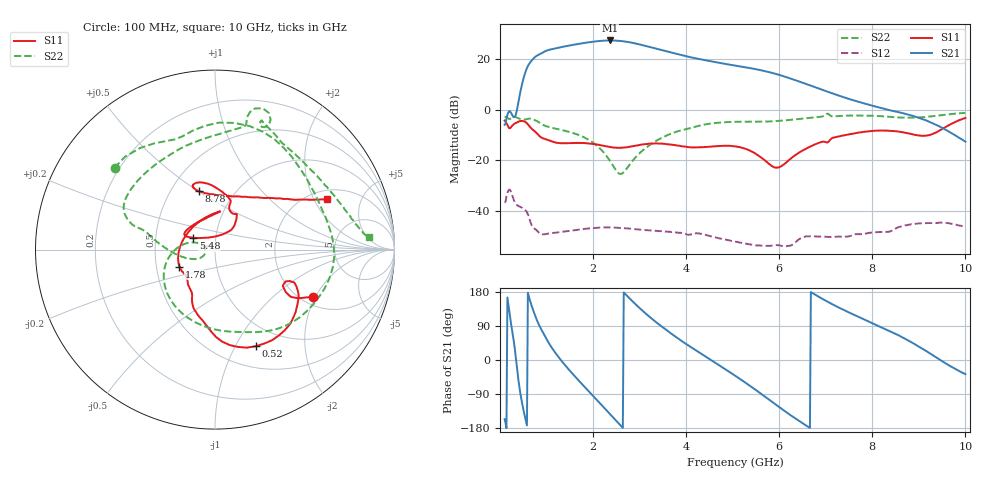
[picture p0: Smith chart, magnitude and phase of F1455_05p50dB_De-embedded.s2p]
! Integrated Device Technology
! Corporate Headquarters
! 6024 Silver Creek Valley Road
! San Jose, CA 95138  USA
! Phone:  1-408-284-8200
! Toll Free:  1-800-223-1366
! Webpage:  http://www.idt.com/
! Timing and RF Division
! 515 Groton Road, Suite 102
! Westford, MA 01886-6024
! Device:  F1455
! Description: 6-bit 0.5 dB Transmit Variable Gain Amplifier
! Frequency:  1400.0 -  2300.00 MHz
! Package:  6x6 mm Thin QFN Plastic Package: 28 pin
! State:  11
! Atten State:  5.5 dB
! Voltage:  +5.00 Volts
! Current:  216.788 mA
! Data:  The device was measured on a the F1455 evaluation board which has
!  individual transmission lines to the RF pins.  Data was collected
!  using a calibrated network analyzer.  The evaluation board was
!  de-embedded using a TRL calibration technique.
!  The reference plane is the edge of the package pin.
!  Pin  1 = CSb
!  Pin  2 = DATA
!  Pin  3 = CLK
!  Pin  4 = RSET
!  Pin  5 = GND
!  Pin  6 = RFIN  = Port 1
!  Pin  7 = GND
!  Pin  8 = NC
!  Pin  9 = NC
!  Pin 10 = NC
!  Pin 11 = NC
!  Pin 12 = NC
!  Pin 13 = NC
!  Pin 14 = /STBY
!  Pin 15 = GND
!  Pin 16 = RFOUT  = Port 2
!  Pin 17 = GND
!  Pin 18 = NC
!  Pin 19 = NC
!  Pin 20 = NC
!  Pin 21 = GND
!  Pin 22 = NC
!  Pin 23 = GND
!  Pin 24 = NC
!  Pin 25 = NC
!  Pin 26 = NC
!  Pin 27 = GND
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# GHz S dB R 50
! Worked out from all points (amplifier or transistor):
!   496 points, 100 MHz to 10 GHz, reference 50 ohm
!   highest |S21| = 27.3 dB at 2.36 GHz (marker M1)
!   |S21| within 3 dB of that: 1.221 GHz to 3.307 GHz (2.086 GHz wide, 92.1 % of centre)
!   unconditionally stable (mu >= 1): start of sweep to end of sweep
!   at 1.74 GHz: K = 4.93, MAG = 26.8 dB, |S12| = -47.2 dB
!   at 5.06 GHz: K = 17.71, MAG = 19.3 dB, |S12| = -52.1 dB
!   at 10 GHz: K = 59.84, MAG = -4.0 dB, |S12| = -46.2 dB
!   S11 on the Smith chart (normalised r, x): 100 MHz: 2.29, -1.92; 520 MHz: 0.74, -1.22; 1.78 GHz: 0.66, -0.13; 5.48 GHz: 0.78, +0.10; 8.78 GHz: 0.68, +0.50; 10 GHz: 2.38, +2.54
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0.1  -4.33 -25.8  -6.01 -156.3  -36.74 41.9  -2.83 140.9
0.38  -4.90 -37.9  1.23 -36.3  -37.89 -108.7  -3.30 55.9
0.52  -4.67 -67.0  13.24 -140.4  -39.32 -154.2  -3.93 24.4
0.7  -7.87 -99.3  19.76 136.1  -46.29 151.3  -3.77 -19.5
0.82  -9.94 -113.6  21.56 97.5  -48.28 135.8  -4.79 -47.9
0.96  -11.56 -120.5  22.94 64.4  -49.21 123.6  -6.33 -72.2
1.14  -12.70 -131.6  23.97 27.6  -48.72 101.0  -7.28 -97.2
1.34  -13.26 -137.7  24.77 -4.9  -48.24 79.2  -8.11 -121.0
1.76  -13.15 -153.5  26.16 -63.2  -47.19 43.8  -10.53 -160.4
1.78  -13.17 -154.5  26.22 -65.8  -47.14 42.3  -10.70 -162.1
2.08  -13.76 -173.4  26.99 -105.1  -46.65 21.4  -14.20 174.1
2.36  -14.75 158.6  27.30 -142.3  -46.50 3.2  -20.14 159.2
2.62  -15.06 126.2  27.05 -176.5  -46.72 -12.2  -25.30 -167.6
2.92  -14.20 97.0  26.08 146.3  -47.24 -27.2  -18.70 -153.6
3.4  -13.38 82.5  23.86 95.5  -47.94 -46.7  -11.91 -178.8
4.1  -14.90 109.4  20.66 34.2  -49.26 -69.9  -7.27 164.4
5.06  -14.51 154.3  17.38 -42.0  -52.15 -106.5  -4.82 148.9
5.48  -17.25 151.3  16.02 -77.6  -53.51 -112.6  -4.78 133.4
6.7  -14.31 53.5  9.32 177.7  -50.01 -143.2  -3.20 78.5
8.36  -8.34 108.1  -0.19 76.9  -48.20 163.9  -2.82 62.4
8.78  -9.45 105.7  -2.02 51.0  -45.47 150.1  -3.18 47.1
10  -3.30 24.5  -12.64 -37.3  -46.24 77.9  -1.30 4.6
